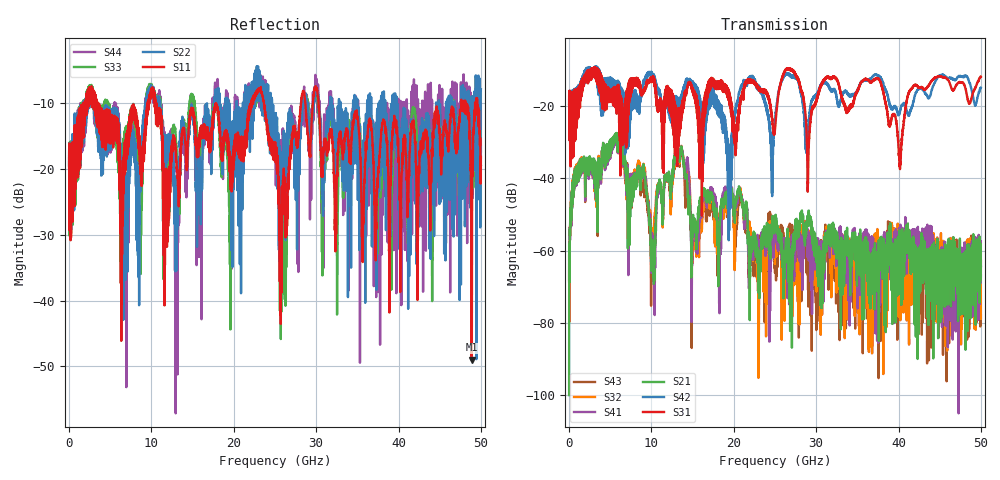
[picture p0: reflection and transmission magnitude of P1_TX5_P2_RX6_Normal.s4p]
!Keysight Technologies,N5225B,MY57041031,A.13.20.10
!Date: Friday, May 31, 2019 11:37:08
!Correction: S11(Full 4 Port(1,2,3,4))
!S12(Full 4 Port(1,2,3,4))
!S13(Full 4 Port(1,2,3,4))
!S14(Full 4 Port(1,2,3,4))
!S21(Full 4 Port(1,2,3,4))
!S22(Full 4 Port(1,2,3,4))
!S23(Full 4 Port(1,2,3,4))
!S24(Full 4 Port(1,2,3,4))
!S31(Full 4 Port(1,2,3,4))
!S32(Full 4 Port(1,2,3,4))
!S33(Full 4 Port(1,2,3,4))
!S34(Full 4 Port(1,2,3,4))
!S41(Full 4 Port(1,2,3,4))
!S42(Full 4 Port(1,2,3,4))
!S43(Full 4 Port(1,2,3,4))
!S44(Full 4 Port(1,2,3,4))
!S4P File: Measurements: <S11,S12,S13,S14>,
!<S21,S22,S23,S24>,
!<S31,S32,S33,S34>,
!<S41,S42,S43,S44>:
# Hz S  dB  R 50.0
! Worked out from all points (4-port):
!   5000 points, 10 MHz to 50 GHz, reference 50 ohm
!   strongest paths, dB at 10 MHz, 12.51 GHz, 25.01 GHz, 37.51 GHz, 50 GHz:
!     S31: -19.3, -23.0, -26.1, -12.3, -11.7
!     S42: -19.4, -16.9, -23.8, -11.4, -14.8
!     S21: -100.1, -39.2, -51.7, -62.2, -64.3
!     S41: -68.5, -39.5, -54.1, -61.1, -66.9
!     S32: -61.4, -40.4, -61.6, -56.0, -78.8
!     S43: -68.0, -39.7, -66.2, -60.0, -62.8
!   lowest |S11| = -49.0 dB at 48.87 GHz (marker M1), VSWR 1.01, Z = 49.7 + j0.133 ohm
!   |S11| at or under -10 dB: 3.502 GHz to 9.556 GHz (6.054 GHz wide, 92.7 % of centre); 10.5 GHz to 22.11 GHz (11.6 GHz wide, 71.2 % of centre); 30.29 GHz to 47.6 GHz (17.31 GHz wide, 44.4 % of centre)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
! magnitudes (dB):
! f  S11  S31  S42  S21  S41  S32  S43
! 10 MHz  -19.9  -19.3  -19.4  -100.1  -68.5  -61.4  -68.0
! 5.6 GHz  -14.4  -18.0  -13.8  -28.1  -28.4  -28.0  -28.0
! 10.19 GHz  -8.2  -12.1  -11.1  -64.9  -60.1  -56.6  -62.8
! 13.1 GHz  -19.8  -22.3  -19.9  -30.7  -31.2  -31.6  -32.2
! 23.02 GHz  -8.1  -15.5  -14.3  -64.0  -62.7  -71.9  -69.4
! 48.87 GHz  -49.0  -17.6  -15.4  -64.8  -68.1  -60.5  -71.3
! 50 GHz  -18.2  -11.7  -14.8  -64.3  -66.9  -78.8  -62.8
